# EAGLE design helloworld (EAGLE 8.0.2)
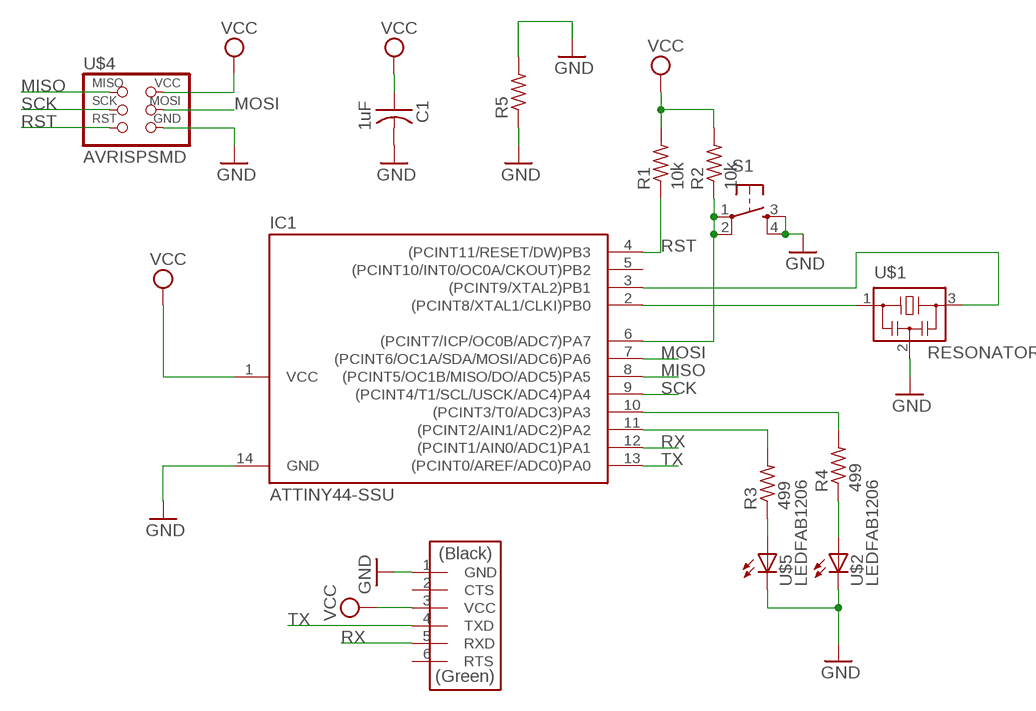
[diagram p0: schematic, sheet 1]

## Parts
C1  1uF  CAP-US1206FAB  [C1206FAB]
IC1  ATTINY44-SSU  [SOIC14]
R1  10k  RES-US1206FAB  [R1206FAB]
R2  10k  RES-US1206FAB  [R1206FAB]
R3  499  RES-US1206FAB  [R1206FAB]
R4  499  RES-US1206FAB  [R1206FAB]
R5  RES-US1206FAB  [R1206FAB]
S1  6MM_SWITCH6MM_SWITCH  [6MM_SWITCH]
U$1  RESONATOR  [EFOBM]
U$2  LEDFAB1206  [LED1206FAB]
U$3  FTDI-SMD-HEADER  [1X06SMD]
U$4  AVRISPSMD  [2X03SMD]
U$5  LEDFAB1206  [LED1206FAB]

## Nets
GND: C1.2 IC1.14(GND) R5.1 R5.2 S1.3(S) S1.4(S1) U$1.2 U$2.2(C) U$3.1(GND) U$4.6(GND) U$5.2(C)
MISO: IC1.8((PCINT5/OC1B/MISO/DO/ADC5)PA5) U$4.1(MISO)
MOSI: IC1.7((PCINT6/OC1A/SDA/MOSI/ADC6)PA6) U$4.4(MOSI)
N$1: IC1.2((PCINT8/XTAL1/CLKI)PB0) U$1.1
N$2: IC1.3((PCINT9/XTAL2)PB1) U$1.3
N$4: IC1.6((PCINT7/ICP/OC0B/ADC7)PA7) R2.1 S1.1(P) S1.2(P1)
N$5: R4.1 U$2.1(A)
N$6: R3.1 U$5.1(A)
N$7: IC1.11((PCINT2/AIN1/ADC2)PA2) R3.2
N$8: IC1.10((PCINT3/T0/ADC3)PA3) R4.2
RST: IC1.4((PCINT11/RESET/DW)PB3) R1.1 U$4.5(RST)
RX: IC1.12((PCINT1/AIN0/ADC1)PA1) U$3.5(RXD)
SCK: IC1.9((PCINT4/T1/SCL/USCK/ADC4)PA4) U$4.3(SCK)
TX: IC1.13((PCINT0/AREF/ADC0)PA0) U$3.4(TXD)
VCC: C1.1 IC1.1(VCC) R1.2 R2.2 U$3.3(VCC) U$4.2(VCC)
Unconnected: IC1.5((PCINT10/INT0/OC0A/CKOUT)PB2) U$3.2(CTS) U$3.6(RTS)

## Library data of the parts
C1 = fab:CAP-US
IC1 = fab:ATTINY44
R1-R5 = fab:RES-US: Resistor (US Symbol)
S1 = fab:6MM_SWITCH: OMRON SWITCH
U$1 = fab:RESONATOR
U$2 U$5 = fab:LED: LED
U$3 = fab:FTDI-SMD-HEADER
U$4 = fab:AVRISP

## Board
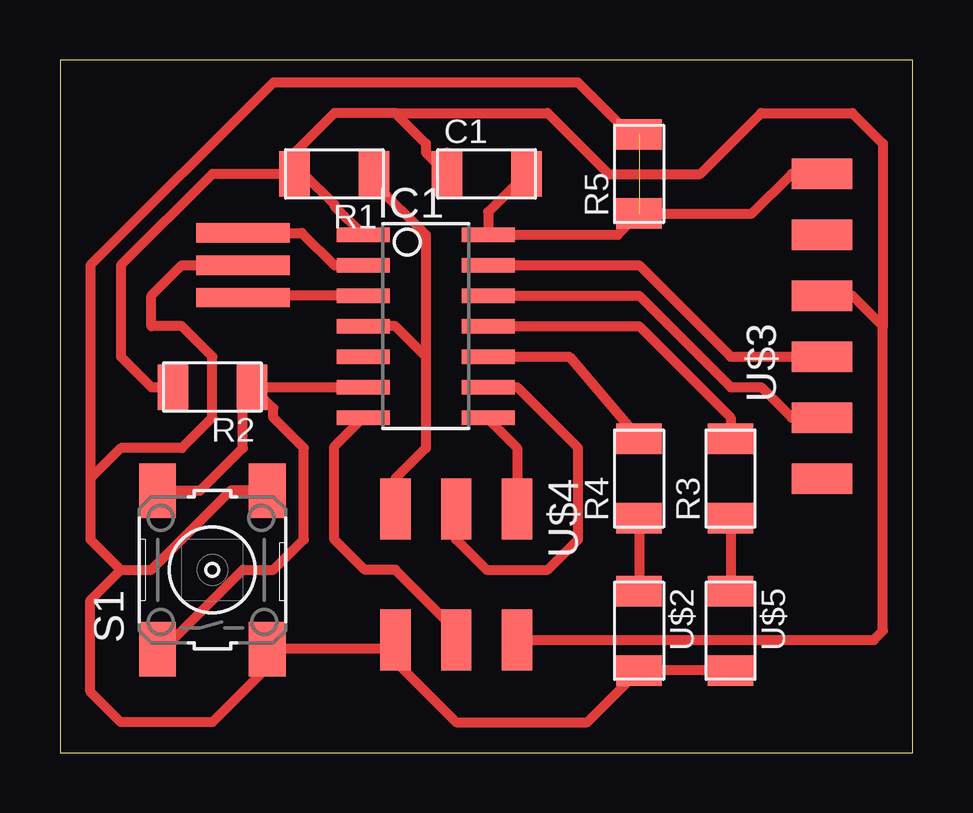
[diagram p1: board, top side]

Size 35.54 x 28.88 mm. Coordinates in mm from the lower left corner, seen from the top.
Outline: 0,0 35.54,0 35.54,28.88 0,28.88 0,0
Copper layers (1*16): Top 0.035mm / dielectric 1.5mm / Bottom 0.035mm
Design rules "default": minimum track width 10mil, minimum drill 24mil, track to track 8mil, track to pad 8mil, pad to pad 8mil, via to via 8mil, smd to smd 8mil, copper to edge 40mil, drill to drill 8mil, minimum pad ring 10mil, minimum via ring 8mil, stop-mask expansion 4mil, vias tented up to drill 0mil, thermal gap 10mil

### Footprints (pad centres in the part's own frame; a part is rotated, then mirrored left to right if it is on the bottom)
C1206FAB = smd 1.27 x 1.905: 1 -1.651,0; 2 1.651,0
SOIC14 = smd 0.61 x 2.21: 1 -3.81,-2.603; 2 -2.54,-2.603; 3 -1.27,-2.603; 4 0,-2.603; 5 1.27,-2.603; 6 2.54,-2.603; 7 3.81,-2.603; 8 3.81,2.603; 9 2.54,2.603; 10 1.27,2.603; 11 0,2.603; 12 -1.27,2.603; 13 -2.54,2.603; 14 -3.81,2.603
R1206FAB = smd 1.27 x 1.905: 1 -1.651,0; 2 1.651,0
6MM_SWITCH = smd 2.286 x 1.524: 1 -3.302,2.286; 2 3.302,2.286; 3 -3.302,-2.286; 4 3.302,-2.286
EFOBM = smd 0.8 x 3.9: 1 -1.35,0; 2 0,0; 3 1.35,0
LED1206FAB = smd 1.27 x 1.905: 1 -1.651,0; 2 1.651,0
1X06SMD = smd 2.54 x 1.27: 1 0,6.35; 2 0,3.81; 3 0,1.27; 4 0,-1.27; 5 0,-3.81; 6 0,-6.35
2X03SMD = smd 2.54 x 1.27: 1 -2.54,2.54; 2 2.92,2.54; 3 -2.54,0; 4 2.92,0; 5 -2.54,-2.54; 6 2.92,-2.54

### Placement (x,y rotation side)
C1  17.78,24.13 0 top
IC1  15.24,17.78 270 top
R1  11.43,24.13 180 top
R2  6.35,15.24 180 top
R3  27.94,11.43 90 top
R4  24.13,11.43 90 top
R5  24.13,24.13 90 top
S1  6.35,7.62 90 top
U$1  7.62,20.32 270 top
U$2  24.13,5.08 270 top
U$3  31.75,17.78 0 top
U$4  16.51,7.62 270 top
U$5  27.94,5.08 270 top

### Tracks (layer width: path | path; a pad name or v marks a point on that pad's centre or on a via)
GND  (1 unrouted)
  Top 0.406: C1.2 17.84,22.54 IC1.14 23.24,21.59 R5.1 28.83,22.48 30.48,24.13 U$3.1 | S1.4 7.11,10.92 3.81,7.62 2.54,7.62 | 2.54,7.62 1.27,8.89 1.27,11.43 | 2.54,7.62 1.27,6.35 1.27,2.54 2.54,1.27 6.35,1.27 8.64,3.56 S1.3 13.59,4.32 U$4.6 13.97,3.81 16.51,1.27 21.97,1.27 U$2.2 U$5.2 | 1.27,11.43 2.54,12.7 5.08,12.7 6.35,13.97 6.35,16.51 5.08,17.78 3.81,17.78 3.81,19.05 5.08,20.32 U$1.2 | R5.2 23.75,25.78 21.59,27.94 8.89,27.94 1.27,20.32 1.27,11.43
MISO
  Top 0.406: IC1.8 17.84,13.91 19.05,12.7 U$4.1
MOSI
  Top 0.406: U$4.4 16.51,5.08 13.97,7.62 12.7,7.62 11.43,8.89 11.43,12.76 IC1.7
N$1
  Top 0.406: U$1.1 10.08,21.67 11.43,20.32 IC1.2
N$2
  Top 0.406: IC1.3 7.7,19.05 U$1.3
N$4
  Top 0.406: 3.81,11.18 S1.2 5.84,10.92 7.62,12.7 7.62,14.86 R2.1 | R2.1 IC1.6 | S1.1 4.32,4.32 7.62,7.62 8.89,7.62 10.16,8.89 10.16,12.7 8.89,13.97 8.89,14.35 R2.1
N$5
  Top 0.406: R4.1 U$2.1
N$6
  Top 0.406: R3.1 U$5.1
N$7
  Top 0.406: IC1.11 24.13,17.78 27.94,13.97 R3.2
N$8
  Top 0.406: IC1.10 21.21,16.51 R4.2
RST
  Top 0.406: U$4.5 13.97,11.43 15.24,12.7 15.24,16.51 | 15.24,16.51 13.97,17.78 IC1.4 | R1.1 13.08,23.75 15.24,21.59 15.24,16.51
RX
  Top 0.406: U$3.5 30.48,13.97 29.21,15.24 27.94,15.24 24.13,19.05 IC1.12
SCK
  Top 0.406: U$4.3 16.51,8.89 17.78,7.62 20.32,7.62 21.59,8.89 21.59,12.7 19.05,15.24 IC1.9
TX
  Top 0.406: U$3.4 27.94,16.51 24.13,20.32 IC1.13
VCC
  Top 0.406: R1.2 10.16,24.13 11.43,22.86 11.43,22.8 IC1.1 | U$4.2 33.91,4.7 34.29,5.08 34.29,17.78 | 34.29,17.78 33.02,19.05 U$3.3 | R1.2 6.35,24.13 2.54,20.32 2.54,16.51 3.81,15.24 R2.2 | 16.13,25.02 C1.1 15.24,25.02 15.24,25.4 13.97,26.67 | 34.29,17.78 34.29,25.4 33.02,26.67 29.21,26.67 26.67,24.13 22.86,24.13 20.32,26.67 13.97,26.67 | R1.2 9.78,25.02 11.43,26.67 13.97,26.67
